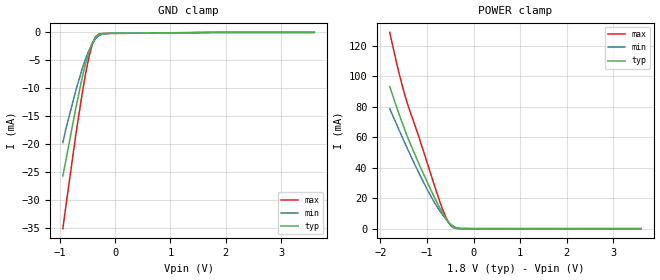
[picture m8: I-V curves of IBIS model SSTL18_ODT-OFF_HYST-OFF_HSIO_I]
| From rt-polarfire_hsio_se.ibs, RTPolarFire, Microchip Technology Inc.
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|   Model SSTL18_ODT-OFF_HYST-OFF_HSIO_I
[Model]   SSTL18_ODT-OFF_HYST-OFF_HSIO_I
Model_type   Input
Vinl =   0.775
Vinh =   1.025
|   typ   min   max
C_comp_pullup   1.335e-12   1.335e-12   1.380e-12
C_comp_pulldown  1.335e-12   1.335e-12   1.380e-12
[Temperature Range]  25C   125C   -55C
[Voltage Range]  1.8   1.71   1.89
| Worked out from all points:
|   GND clamp passes 1 mA (typ) near -0.36 V on its own axis
|   POWER clamp passes 1 mA (typ) near -0.43 V on its own axis
[GND Clamp]
| Voltage   I(typ)   I(min)   I(max)
-945mV    -25.64mA   -19.68mA   -35.03mA
-885.9mV  -22.62mA   -17.06mA   -30.7mA
-708.7mV  -13.41mA   -10.29mA   -18.16mA
-590.6mV  -7.869mA   -6.334mA   -10.59mA
-531.6mV  -5.486mA   -4.627mA   -7.255mA
-472.5mV  -3.471mA   -3.166mA   -4.373mA
-413.4mV  -1.919mA   -1.995mA   -2.137mA
-354.4mV  -899.8uA   -1.144mA   -780.3uA
-295.3mV  -390.3uA   -603uA     -297.2uA
-236.2mV  -211.8uA   -316uA     -206.4uA
-59.06mV  -146uA     -127.3uA   -182.2uA
3.6V      0A         0A         0A
[POWER Clamp]
| Voltage   I(typ)   I(min)   I(max)
-1.8V     93.14mA    78.64mA    128.6mA
-1.595V   74.67mA    64.33mA    101.3mA
-1.417V   60.1mA     52.26mA    81.76mA
-1.181V   43.1mA     36.95mA    60.82mA
-1.004V   31.09mA    26.19mA    43.97mA
-708.7mV  12.66mA    10.93mA    16.36mA
-590.6mV  6.471mA    6.139mA    7.229mA
-531.6mV  3.924mA    4.133mA    3.799mA
-472.5mV  1.945mA    2.472mA    1.513mA
-354.4mV  180.5uA    510.3uA    87.9uA
-59.06mV  7.629uA    10.67uA    9.815uA
3.6V      0A         0A         0A
